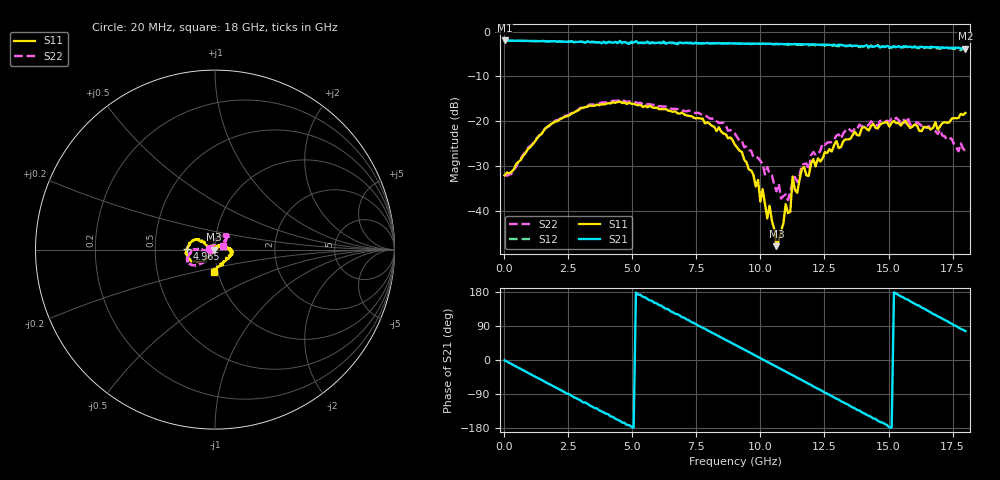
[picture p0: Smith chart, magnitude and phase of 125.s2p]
!Agilent Technologies,N5230A,US43500223,A.07.50.48
!Agilent N5230A: A.07.50.48
!Date: Saturday, January 16, 2016 15:57:35
!Correction: S11(Full 2 Port(1,2))
!S21(Full 2 Port(1,2))
!S12(Full 2 Port(1,2))
!S22(Full 2 Port(1,2))
!S2P File: Measurements: S11, S21, S12, S22:
# Hz S  dB  R 50
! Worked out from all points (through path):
!   201 points, 20 MHz to 18 GHz, reference 50 ohm
!   highest |S21| = -1.98 dB at 20 MHz (marker M1); lowest = -3.8 dB at 18 GHz (marker M2)
!   group delay of S21, straight-line fit = 99.1 ps
!   lowest |S11| = -47.9 dB at 10.63 GHz (marker M3), VSWR 1.01, Z = 49.6 - j0.0615 ohm
!   |S11| at or under -10 dB: start of sweep to end of sweep
!   |S22| runs from -37.6 to -15.3 dB; largest |S21 - S12| = 0.071
!   S11 on the Smith chart (normalised r, x): 20 MHz: 0.95, +0.00; 4.965 GHz: 0.73, +0.01; 18 GHz: 0.96, -0.24
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2e7  -32.07 178.1  -1.98 -0.8  -1.98 -0.9  -31.98 176.2
1.5483e9  -22.06 -134.1  -2.09 -56.0  -2.10 -56.4  -21.99 -127.2
3.0766e9  -16.99 -152.5  -2.32 -111.9  -2.31 -111.8  -17.04 -141.7
4.9645e9  -16.06 178.7  -2.26 -175.8  -2.40 -179.2  -15.62 -161.4
6.0433e9  -17.28 161.0  -2.43 145.0  -2.59 142.5  -16.66 -168.2
7.4817e9  -19.36 148.0  -2.44 94.9  -2.66 92.3  -18.20 -176.5
9.01e9  -25.27 151.9  -2.64 40.3  -2.70 37.6  -22.79 -176.6
9.909e9  -33.11 173.3  -2.69 8.2  -2.77 5.3  -28.14 -169.7
9.9989e9  -37.90 -171.1  -2.69 4.7  -2.77 2.2  -28.84 -158.2
1.00888e10  -35.17 158.2  -2.69 1.6  -2.73 -1.2  -29.46 -160.0
1.02686e10  -41.67 156.8  -2.73 -4.9  -2.80 -7.5  -30.22 -165.5
1.03585e10  -38.84 168.6  -2.72 -8.0  -2.78 -10.9  -31.64 -170.2
1.06282e10  -47.87 -171.2  -2.73 -17.6  -2.78 -20.5  -35.63 -168.1
1.09878e10  -38.49 19.9  -2.81 -30.4  -2.87 -34.1  -36.33 151.6
1.11676e10  -40.18 60.0  -2.80 -36.8  -2.82 -40.1  -35.63 135.8
1.12575e10  -32.33 50.9  -2.83 -40.2  -2.87 -44.1  -33.56 122.4
1.14373e10  -35.97 29.4  -2.81 -46.9  -2.90 -49.6  -33.52 115.4
1.20666e10  -28.44 35.1  -2.82 -69.9  -2.87 -73.1  -26.85 89.6
1.3505e10  -23.93 8.2  -3.01 -121.6  -3.09 -125.3  -21.97 71.9
1.50333e10  -21.17 -8.0  -3.40 -177.9  -3.66 179.4  -20.11 53.0
1.65616e10  -21.44 -55.9  -3.57 129.0  -3.58 123.4  -21.05 43.1
1.8e10  -18.17 -92.9  -3.79 76.3  -3.96 70.0  -26.66 23.5
